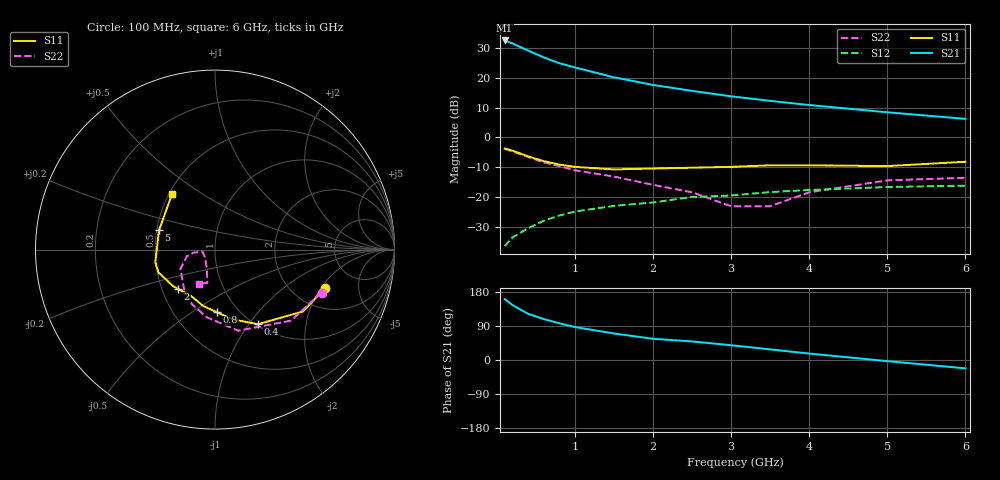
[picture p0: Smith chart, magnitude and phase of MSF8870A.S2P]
!  MSF-8870 S PARAMETERS
!  Id=36mA  LAST UPDATED 07-27-92
# ghz s ma r 50
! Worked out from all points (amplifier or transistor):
!   14 points, 100 MHz to 6 GHz, reference 50 ohm
!   highest |S21| = 32.5 dB at 100 MHz (marker M1)
!   |S21| within 3 dB of that: start of sweep to 368.3 MHz
!   unconditionally stable (mu >= 1): 2.121 GHz to end of sweep
!   at 400 MHz: K = 0.64, MSG = 29.8 dB, |S12| = -30.5 dB
!   at 2 GHz: K = 0.99, MSG = 19.7 dB, |S12| = -21.8 dB
!   at 6 GHz: K = 1.37, MAG = 7.6 dB, |S12| = -16.2 dB
!   S11 on the Smith chart (normalised r, x): 100 MHz: 2.99, -2.19; 400 MHz: 1.03, -1.11; 800 MHz: 0.80, -0.64; 2 GHz: 0.61, -0.29; 5 GHz: 0.51, +0.12; 6 GHz: 0.52, +0.38
0.1  0.65 -19.0  42.04 161.0  0.015 40.0  0.64 -22.0
0.2  0.6 -35.0  37.54 145.0  0.021 47.0  0.58 -43.0
0.4  0.48 -60.0  28.49 122.0  0.03 51.0  0.47 -74.0
0.6  0.4 -76.0  21.9 108.0  0.04 50.0  0.38 -97.0
0.8  0.35 -88.0  17.48 97.0  0.049 50.0  0.33 -113.0
1  0.32 -102.0  14.85 87.0  0.057 51.0  0.28 -128.0
1.5  0.29 -118.0  10.14 70.0  0.071 47.0  0.22 -151.0
2  0.3 -133.0  7.55 56.0  0.081 45.0  0.16 -167.0
2.5  0.31 -139.0  6.01 49.0  0.1 46.0  0.12 -172.0
3  0.32 -149.0  4.87 39.0  0.106 41.0  0.07 -170.0
3.5  0.34 -158.0  4.09 28.0  0.121 35.0  0.07 -143.0
4  0.34 -168.0  3.48 17.0  0.131 31.0  0.12 -112.0
5  0.33 161.0  2.63 -3.0  0.147 21.0  0.19 -103.0
6  0.39 128.0  2.04 -22.0  0.155 10.0  0.21 -115.0
